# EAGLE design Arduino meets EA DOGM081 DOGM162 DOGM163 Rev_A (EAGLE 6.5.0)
Assembly variants: 3.3V monochrome, 5V monochrome, 3.3V RGB, 5V RGB
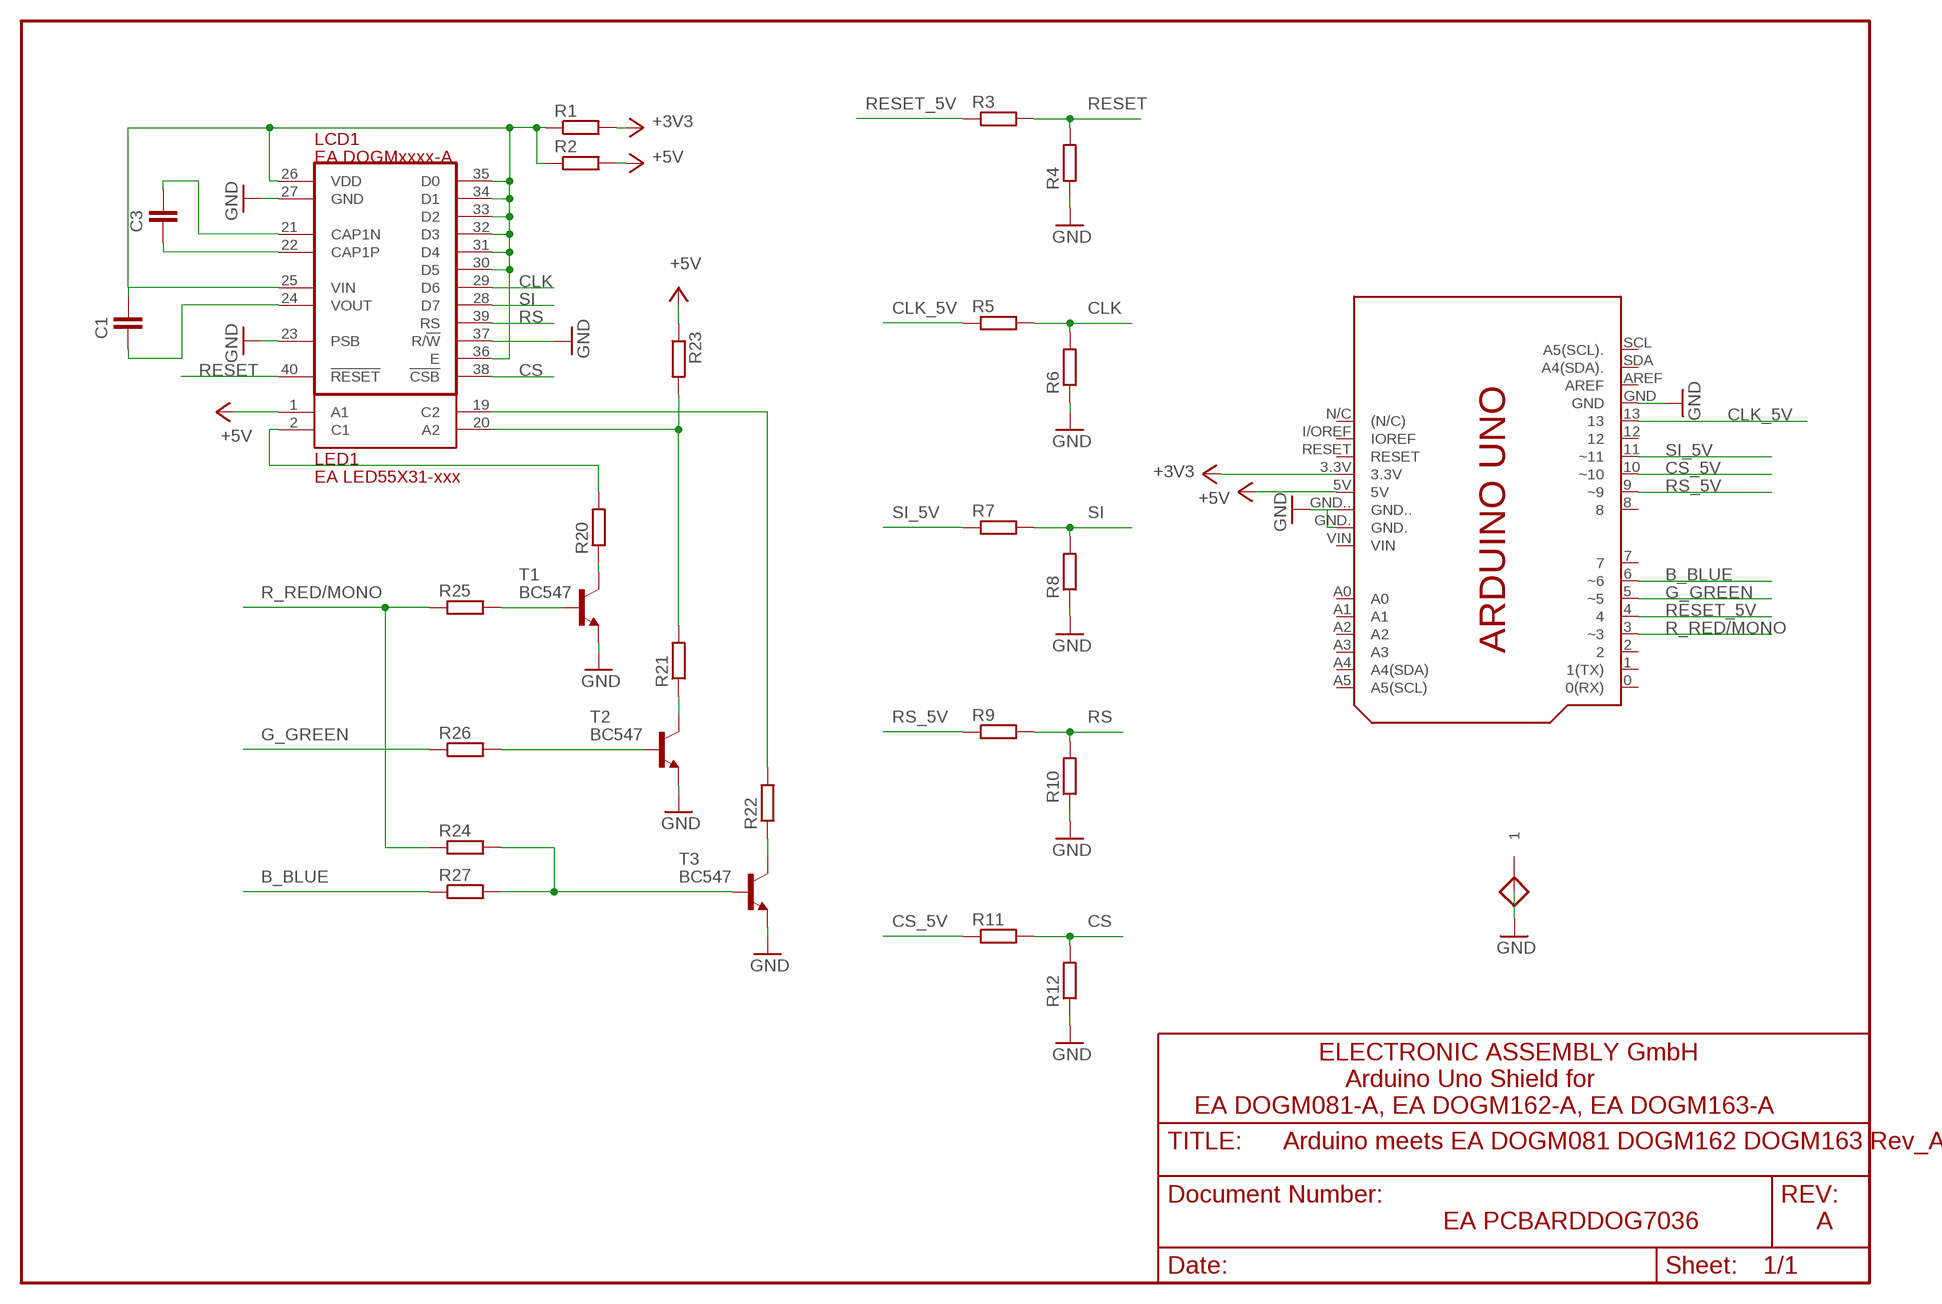
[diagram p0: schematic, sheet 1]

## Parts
C1  1uF  C_5MM_AND_1206  [C_5MM_AND_1206]  (not fitted in variant 5V monochrome)  (not fitted in variant 5V RGB)
C3  1uF  C_5MM_AND_1206  [C_5MM_AND_1206]  (not fitted in variant 5V monochrome)  (not fitted in variant 5V RGB)
GND  PAD55/35  [PAD55/35]
LCD1  EA DOGMxxxx-A  EA_DOGM162  [EA_DOGM]
LED1  EA LED55X31-xxx  EA_LED55X31_MONO  [EA_LED55X31]
PCB1  ARDUINO_UNO_SHIELD  [ARDUINO_UNO_SHIELD]
R1  0R  R_10MM_AND_1206  [R_10MM_AND_1206]  (not fitted in variant 5V monochrome)  (not fitted in variant 5V RGB)
R2  0R  R_10MM_AND_1206  [R_10MM_AND_1206]  (not fitted in variant 3.3V monochrome)  (not fitted in variant 3.3V RGB)
R3  2k7  R_10MM_AND_1206  [R_10MM_AND_1206]
R4  4k7  R_10MM_AND_1206  [R_10MM_AND_1206]  (not fitted in variant 5V monochrome)  (not fitted in variant 5V RGB)
R5  2k7  R_10MM_AND_1206  [R_10MM_AND_1206]
R6  4k7  R_10MM_AND_1206  [R_10MM_AND_1206]  (not fitted in variant 5V monochrome)  (not fitted in variant 5V RGB)
R7  2k7  R_10MM_AND_1206  [R_10MM_AND_1206]
R8  4k7  R_10MM_AND_1206  [R_10MM_AND_1206]  (not fitted in variant 5V monochrome)  (not fitted in variant 5V RGB)
R9  2k7  R_10MM_AND_1206  [R_10MM_AND_1206]
R10  4k7  R_10MM_AND_1206  [R_10MM_AND_1206]  (not fitted in variant 5V monochrome)  (not fitted in variant 5V RGB)
R11  2k7  R_10MM_AND_1206  [R_10MM_AND_1206]
R12  4k7  R_10MM_AND_1206  [R_10MM_AND_1206]  (not fitted in variant 5V monochrome)  (not fitted in variant 5V RGB)
R20  R_10MM_AND_1206  [R_10MM_AND_1206]
R21  R_10MM_AND_1206  [R_10MM_AND_1206]  (not fitted in variant 3.3V monochrome)  (not fitted in variant 5V monochrome)
R22  R_10MM_AND_1206  [R_10MM_AND_1206]
R23  0R  R_10MM_AND_1206  [R_10MM_AND_1206]  (not fitted in variant 3.3V RGB)  (not fitted in variant 5V RGB)
R24  470R  R_10MM_AND_1206  [R_10MM_AND_1206]  (not fitted in variant 3.3V RGB)  (not fitted in variant 5V RGB)
R25  470R  R_10MM_AND_1206  [R_10MM_AND_1206]
R26  470R  R_10MM_AND_1206  [R_10MM_AND_1206]  (not fitted in variant 3.3V monochrome)  (not fitted in variant 5V monochrome)
R27  470R  R_10MM_AND_1206  [R_10MM_AND_1206]  (not fitted in variant 3.3V monochrome)  (not fitted in variant 5V monochrome)
T1  BC547  [TO92]
T2  BC547  [TO92]  (not fitted in variant 3.3V monochrome)  (not fitted in variant 5V monochrome)
T3  BC547  [TO92]

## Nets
+3V3: PCB1.3.3V R1.2
+5V: LED1.1(A1) PCB1.5V R2.2 R23.1
B_BLUE: PCB1.6(~6) R27.1
CLK: LCD1.29(D6) R5.2 R6.2
CLK_5V: PCB1.13 R5.1
CS: LCD1.38(!CSB!) R11.2 R12.2
CS_5V: PCB1.10(~10) R11.1
G_GREEN: PCB1.5(~5) R26.1
GND: GND.1 LCD1.23(PSB) LCD1.27(GND) LCD1.37(R/!W!) PCB1.GND PCB1.GND. PCB1.GND.. R4.1 R6.1 R8.1 R10.1 R12.1 T1.1(E) T2.1(E) T3.1(E)
N$6: R20.1 T1.3(C)
N$7: LED1.2(C1) R20.2
N$8: R26.2 T2.2(B)
N$9: C3.2 LCD1.21(CAP1N)
N$10: C3.1 LCD1.22(CAP1P)
N$11: C1.1 LCD1.24(VOUT)
N$12: R25.2 T1.2(B)
N$13: LED1.20(A2) R21.2 R23.2
N$14: LED1.19(C2) R22.2
N$15: R21.1 T2.3(C)
N$16: R22.1 T3.3(C)
N$17: R24.2 R27.2 T3.2(B)
R_RED/MONO: PCB1.3(~3) R24.1 R25.1
RESET: LCD1.40(!RESET!) R3.2 R4.2
RESET_5V: PCB1.4 R3.1
RS: LCD1.39(RS) R9.2 R10.2
RS_5V: PCB1.9(~9) R9.1
SI: LCD1.28(D7) R7.2 R8.2
SI_5V: PCB1.11(~11) R7.1
VDD_LCD: C1.2 LCD1.25(VIN) LCD1.26(VDD) LCD1.30(D5) LCD1.31(D4) LCD1.32(D3) LCD1.33(D2) LCD1.34(D1) LCD1.35(D0) LCD1.36(E) R1.1 R2.1
Unconnected: PCB1.0(0(RX)) PCB1.1(1(TX)) PCB1.2 PCB1.7 PCB1.8 PCB1.12 PCB1.A0 PCB1.A1 PCB1.A2 PCB1.A3 PCB1.A4(A4(SDA)) PCB1.A5(A5(SCL)) PCB1.AREF PCB1.I/OREF(IOREF) PCB1.N/C((N/C)) PCB1.RESET PCB1.SCL(A5(SCL).) PCB1.SDA(A4(SDA).) PCB1.VIN

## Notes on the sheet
- ELECTRONIC ASSEMBLY GmbH
- Arduino Uno Shield for
- EA DOGM081-A, EA DOGM162-A, EA DOGM163-A
- EA PCBARDDOG7036 | A

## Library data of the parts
C1 C3 = EA:C_5MM_AND_1206
GND = EA:PAD55/35
LCD1 = EA:EA_DOGM162: ELECTRONIC ASSEMBYL GmbH EA DOGM162-A EA DOGM081-A EA DOGM163-A
LED1 = EA:EA_LED55X31_MONO
PCB1 = E14_Arduino:ARDUINO_UNO_SHIELD
R1-R12 R20-R27 = EA:R_10MM_AND_1206
T1-T3 = transistor-npn:BC547: NPN TRANSISTOR

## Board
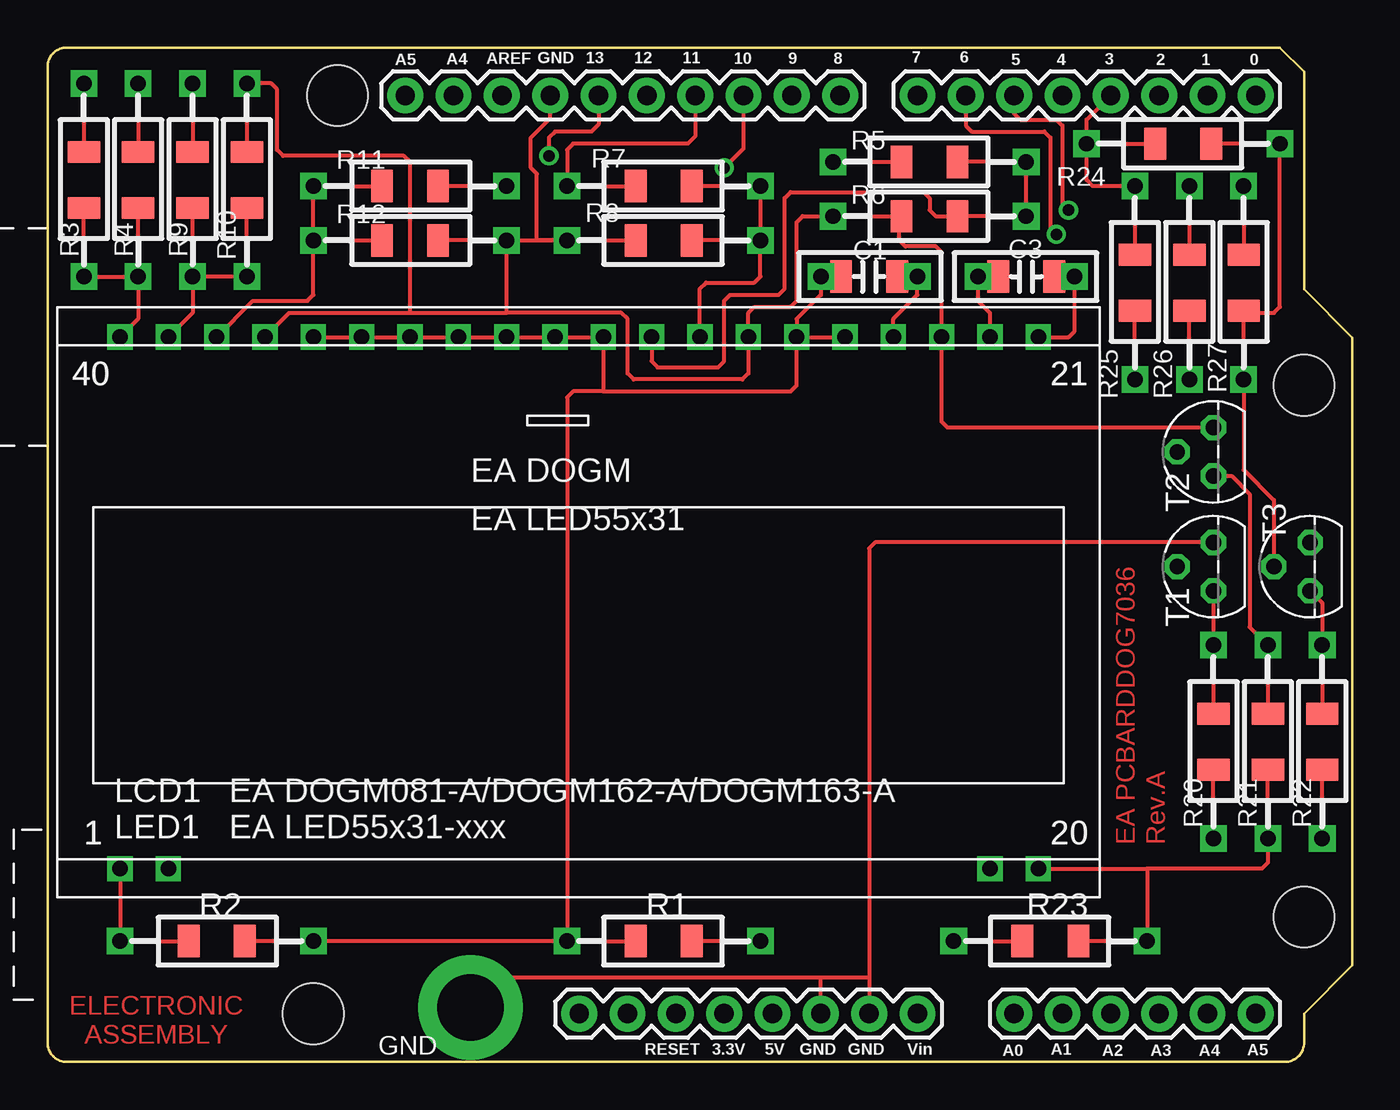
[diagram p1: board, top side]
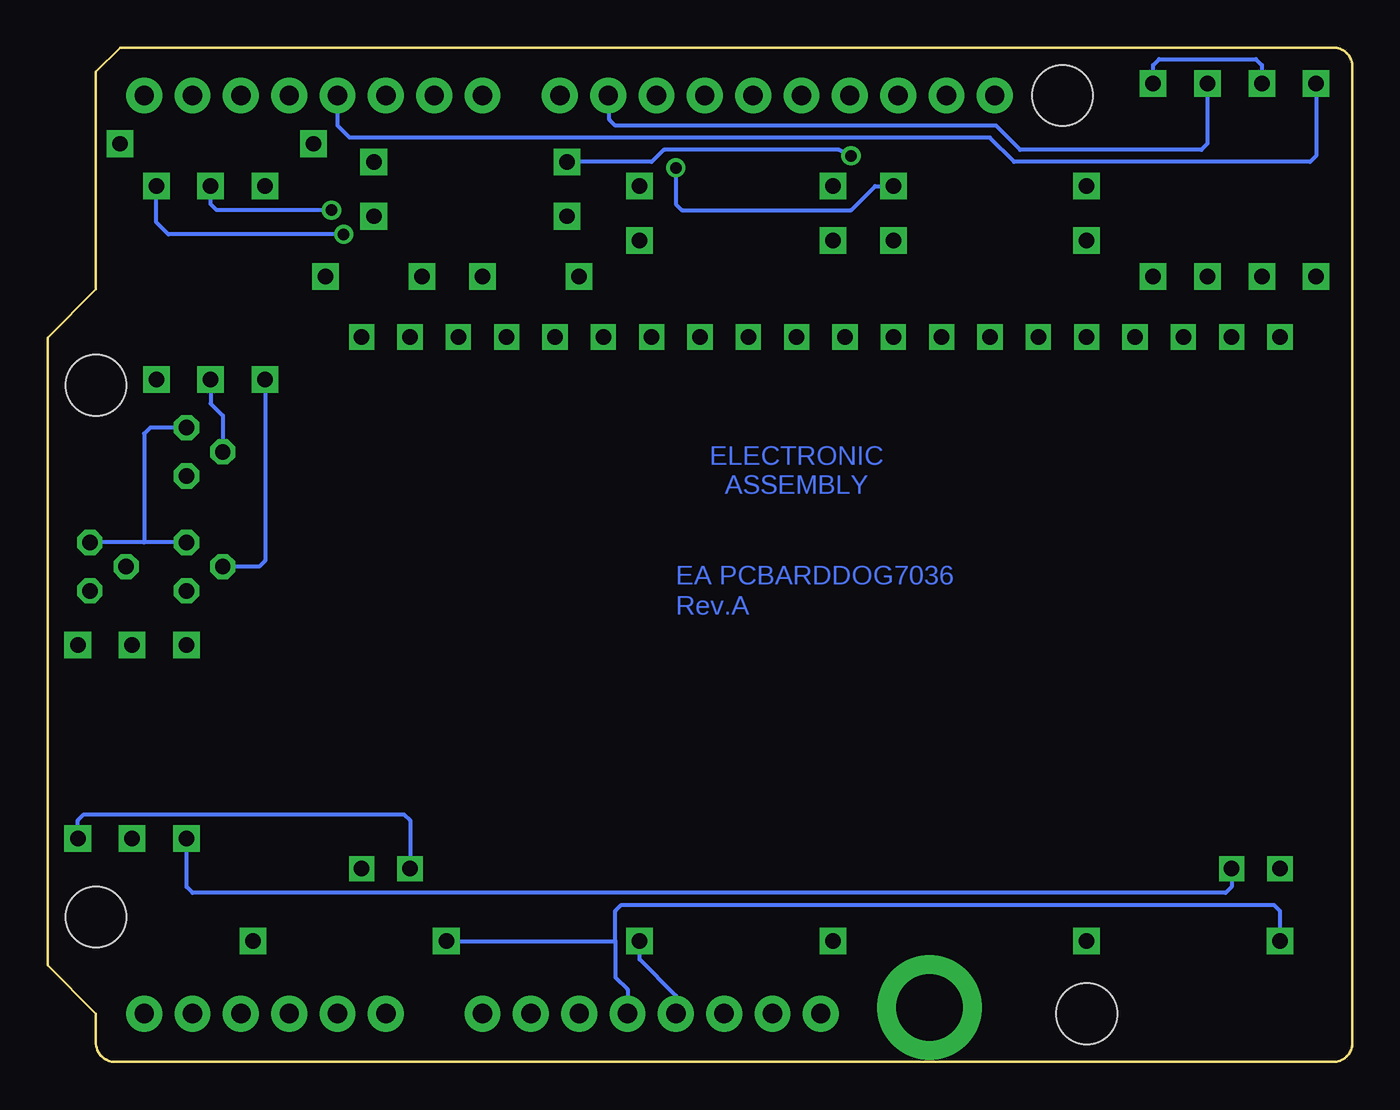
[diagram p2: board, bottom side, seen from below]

Size 68.58 x 53.31 mm. Coordinates in mm from the lower left corner, seen from the top.
Outline: 66.04,2.54 66.04,1.02 arc-90 65.02,0 1.02,0 arc-90 0,1.02 0,52.3 arc-90 1.02,53.31 64.77,53.31 66.04,52.05 66.04,40.62 68.58,38.08 68.58,5.08 66.04,2.54
Copper layers (1*16): Top 0.035mm / dielectric 1.5mm / Bottom 0.035mm
Design rules "default *": minimum track width 8mil, minimum drill 23mil, track to track 8mil, track to pad 8mil, pad to pad 8mil, via to via 8mil, smd to smd 8mil, copper to edge 40mil, drill to drill 8mil, minimum pad ring 10mil, minimum via ring 8mil, stop-mask expansion 4mil, vias tented up to drill 0mil, thermal gap 10mil

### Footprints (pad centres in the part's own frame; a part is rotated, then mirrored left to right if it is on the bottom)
C_5MM_AND_1206 = drill 0.813 pad 1.397 square: 1 0,0; 2 5.08,0 | smd 1.143 x 1.702: 3 4.013,0; 4 1.067,0
PAD55/35 = drill 3.5 pad 5.5: 1 0,0
EA_DOGM = drill 0.813 square: 1 0,0; 2 2.54,0; 19 45.72,0; 20 48.26,0; 21 48.26,27.94; 22 45.72,27.94; 23 43.18,27.94; 24 40.64,27.94; 25 38.1,27.94; 26 35.56,27.94; 27 33.02,27.94; 28 30.48,27.94; 29 27.94,27.94; 30 25.4,27.94; 31 22.86,27.94; 32 20.32,27.94; 33 17.78,27.94; 34 15.24,27.94; 35 12.7,27.94; 36 10.16,27.94; 37 7.62,27.94; 38 5.08,27.94; 39 2.54,27.94; 40 0,27.94
EA_LED55X31 = drill 0.813 square: 1 0,0; 2 2.54,0; 19 45.72,0; 20 48.26,0; 21 48.26,27.94; 22 45.72,27.94; 23 43.18,27.94; 24 40.64,27.94; 25 38.1,27.94; 26 35.56,27.94; 27 33.02,27.94; 28 30.48,27.94; 29 27.94,27.94; 30 25.4,27.94; 31 22.86,27.94; 32 20.32,27.94; 33 17.78,27.94; 34 15.24,27.94; 35 12.7,27.94; 36 10.16,27.94; 37 7.62,27.94; 38 5.08,27.94; 39 2.54,27.94; 40 0,27.94
ARDUINO_UNO_SHIELD = drill 1.016 pad 1.88: 0 63.5,50.8; 1 60.96,50.8; 2 58.42,50.8; 3 55.88,50.8; 3.3V 35.56,2.54; 4 53.34,50.8; 5 50.8,50.8; 5V 38.1,2.54; 6 48.26,50.8; 7 45.72,50.8; 8 41.656,50.8; 9 39.116,50.8; 10 36.576,50.8; 11 34.036,50.8; 12 31.496,50.8; 13 28.956,50.8; A0 50.8,2.54; A1 53.34,2.54; A2 55.88,2.54; A3 58.42,2.54; A4 60.96,2.54; A5 63.5,2.54; AREF 23.876,50.8; GND 26.416,50.8; GND. 43.18,2.54; GND.. 40.64,2.54; I/OREF 30.48,2.54; N/C 27.94,2.54; RESET 33.02,2.54; SCL 18.796,50.8; SDA 21.336,50.8; VIN 45.72,2.54 | hole 3.2: 66.04,7.62; 66.04,35.56; 15.24,50.8; 13.97,2.54
R_10MM_AND_1206 = drill 0.813 pad 1.397 square: 1 0,0; 2 10.16,0 | smd 1.143 x 1.702: 3 6.553,0; 4 3.607,0
TO92 = drill 0.813 octagon: 1 1.27,0; 2 0,1.905; 3 -1.27,0

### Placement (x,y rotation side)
C1  45.72,41.27 180 top
C3  48.9,41.27 0 top
GND  22.23,2.86 0 top
LCD1  3.81,10.16 0 top
LED1  3.81,10.16 0 top
PCB1  0,0 0 top
R1  27.3,6.35 0 top
R2  13.97,6.35 180 top
R3  1.91,51.44 270 top
R4  4.76,51.44 270 top
R5  41.27,47.31 0 top
R6  41.27,44.45 0 top
R7  27.3,46.04 0 top
R8  27.3,43.18 0 top
R9  7.62,51.44 270 top
R10  10.48,51.44 270 top
R11  24.13,46.04 180 top
R12  24.13,43.18 180 top
R20  61.28,21.91 270 top
R21  64.14,21.91 270 top
R22  66.99,21.91 270 top
R23  47.62,6.35 0 top
R24  54.61,48.26 0 top
R25  57.15,46.04 270 top
R26  60.01,46.04 270 top
R27  62.87,46.04 270 top
T1  61.28,26.04 90 top
T2  61.28,32.07 90 top
T3  66.36,26.04 90 top

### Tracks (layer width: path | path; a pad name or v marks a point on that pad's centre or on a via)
+3V3
  Bottom 0.203: PCB1.3.3V 35.56,3.49 37.47,5.4 R1.2
+5V
  Top 0.203: LED1.1 R2.2
  Bottom 0.203: R23.1 38.73,6.35 | 38.73,6.35 38.73,4.45 38.1,3.81 PCB1.5V | 38.73,6.35 38.73,7.94 38.42,8.26 4.13,8.26 3.81,7.94 R2.2
B_BLUE  (via drill 0.6)
  Top 0.203: PCB1.6 48.26,49.21 48.58,48.9 52.39,48.9 52.7,48.58 52.7,43.81 v53.02,43.5
  Bottom 0.203: v53.02,43.5 62.23,43.5 62.87,44.13 R27.1
CLK
  Top 0.203: R6.2 R5.2 | LCD1.29 31.75,36.83 32.07,36.51 35.24,36.51 35.56,36.83 35.56,40.01 35.88,40.32 38.42,40.32 38.73,40.64 38.73,45.4 39.05,45.72 46.04,45.72 46.35,45.4 46.35,44.77 46.67,44.45 48.26,44.45
CLK_5V  (via drill 0.6)
  Top 0.203: PCB1.13 28.96,49.28 28.57,48.9 26.67,48.9 26.35,48.58 v26.35,47.62
  Bottom 0.203: v26.35,47.62 26.99,47.94 36.2,47.94 36.83,47.31 R5.1
CS
  Top 0.203: LCD1.38 10.79,40.01 13.65,40.01 13.97,40.32 R12.2 R11.2
CS_5V  (via drill 0.6)
  Top 0.203: PCB1.10 36.58,48.01 v35.56,46.99
  Bottom 0.203: v35.56,46.99 35.56,45.09 35.24,44.77 26.35,44.77 25.08,46.04 R11.1
G_GREEN  (via drill 0.6)
  Top 0.203: PCB1.5 50.8,49.85 51.12,49.53 53.02,49.53 53.34,49.21 53.34,45.09 v53.66,44.77
  Bottom 0.203: v53.66,44.77 59.69,44.77 60.01,45.09 R26.1
GND
  Top 0.203: LCD1.37 12.7,39.37 19.05,39.37 | 19.05,39.37 24.13,39.37 | 24.13,39.37 R12.1 R8.1 25.72,43.18 25.72,46.67 25.4,46.99 25.4,48.58 26.42,49.59 PCB1.GND | 19.05,39.37 19.05,47.31 18.73,47.62 12.38,47.62 12.06,47.94 12.06,51.12 11.75,51.44 R10.1 | 24.13,39.37 30.16,39.37 30.48,39.05 30.48,36.2 30.8,35.88 36.51,35.88 36.83,36.2 LCD1.27 36.83,39.37 37.15,39.69 39.05,39.69 39.37,40.01 39.37,44.13 39.69,44.45 R6.1 | 44.45,44.45 44.77,44.13 44.77,43.18 45.09,42.86 46.67,42.86 46.99,42.55 LCD1.23 46.99,33.66 47.31,33.34 T2.1 | GND.1 24.45,4.45 40.64,4.45 | PCB1.GND.. 40.64,4.45 | T1.1 43.5,27.3 43.18,26.99 43.18,4.45 | 43.18,4.45 PCB1.GND. | 40.64,4.45 43.18,4.45
  Bottom 0.203: R10.1 10.48,52.39 10.16,52.7 5.08,52.7 4.76,52.39 R4.1 | T1.1 63.5,27.3 | 63.5,27.3 T3.1 | T2.1 63.18,33.34 63.5,33.02 63.5,27.3
N$6
  Top 0.203: T1.3 R20.1
N$7
  Bottom 0.203: LED1.2 6.35,9.21 6.67,8.89 60.96,8.89 61.28,9.21 R20.2
N$8
  Bottom 0.203: R26.2 60.01,34.61 59.37,33.97 T2.2
N$9
  Top 0.203: LCD1.21 53.66,38.1 53.98,38.42 C3.2
N$10
  Top 0.203: C3.1 48.9,40.01 49.53,39.37 LCD1.22
N$11
  Top 0.203: LCD1.24 44.45,39.05 45.72,40.32 C1.1
N$12
  Bottom 0.203: R25.2 57.15,26.35 57.47,26.04 T1.2
N$13
  Top 0.203: R21.2 64.14,10.48 63.82,10.16 57.78,10.16 | LED1.20 57.78,10.16 | 57.78,10.16 R23.2
N$14
  Bottom 0.203: R22.2 66.99,12.7 66.67,13.02 49.85,13.02 49.53,12.7 LED1.19
N$15
  Top 0.203: T2.3 62.23,30.8 63.18,29.84 63.18,22.86 R21.1
N$16
  Top 0.203: T3.3 66.99,24.13 R22.1
N$17
  Top 0.203: 62.87,39.05 62.87,39.37 64.45,39.37 64.77,39.69 R24.2 | R27.2 62.87,31.11 64.45,29.53 T3.2
R_RED/MONO
  Top 0.203: PCB1.3 54.61,49.53 R24.1 54.61,46.35 54.93,46.04 R25.1
RESET
  Top 0.203: R3.2 R4.2 4.76,39.05 LCD1.40
RESET_5V
  Bottom 0.203: R3.1 1.91,47.62 2.22,47.31 17.78,47.31 19.05,48.58 52.7,48.58 53.34,49.21 PCB1.4
RS
  Top 0.203: R10.2 R9.2 7.62,39.37 LCD1.39
RS_5V
  Bottom 0.203: R9.1 7.62,48.26 7.94,47.94 17.46,47.94 18.73,49.21 38.73,49.21 39.05,49.53 39.05,50.74 PCB1.9
SI
  Top 0.203: R7.2 R8.2 37.47,41.27 37.15,40.96 34.61,40.96 34.29,40.64 LCD1.28
SI_5V
  Top 0.203: PCB1.11 34.04,48.64 33.66,48.26 27.62,48.26 27.3,47.94 R7.1
VDD_LCD
  Top 0.203: LCD1.36 LCD1.35 LCD1.34 LCD1.33 LCD1.32 LCD1.31 LCD1.30 29.21,35.24 | 29.21,35.24 39.05,35.24 39.37,35.56 LCD1.26 | LCD1.26 LCD1.25 | C1.2 40.64,40.32 39.37,39.05 LCD1.26 | R2.1 R1.1 27.3,34.92 27.62,35.24 29.21,35.24

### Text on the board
Top: EA PCBARDDOG7036 | Rev.A | ELECTRONIC / ASSEMBLY
Bottom: ELECTRONIC / ASSEMBLY | EA PCBARDDOG7036 | Rev.A
tPlace: EA DOGM081-A/DOGM162-A/DOGM163-A | EA LED55x31-xxx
